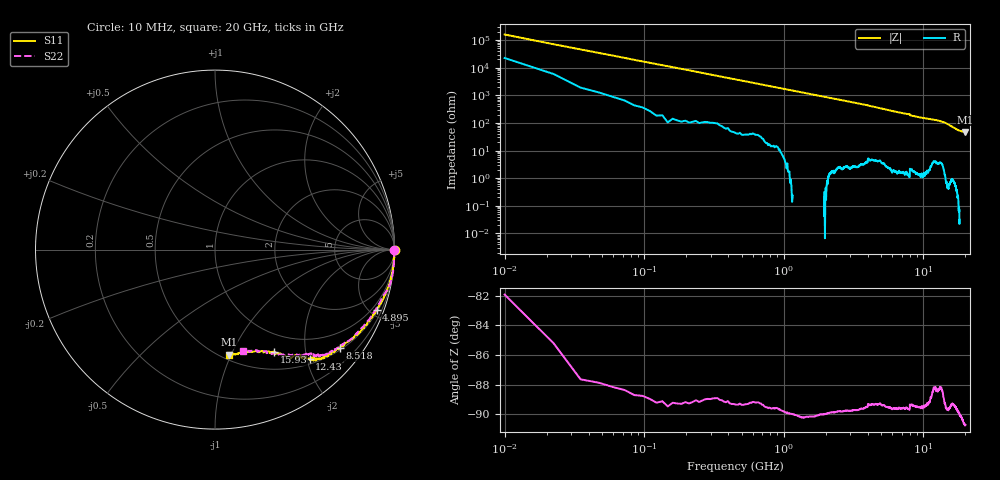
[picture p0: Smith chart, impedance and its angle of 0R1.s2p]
!Keysight Technologies,P5008B,MY61100088,A.16.20.02
!Date: Monday, May 27, 2024 12:57:32
!Correction: S11(C  2-Port  )
!S21(C  2-Port  )
!S12(C  2-Port  )
!S22(C  2-Port  )
!S2P File: Measurements: S11, S21, S12, S22:
# Hz S  dB  R 50
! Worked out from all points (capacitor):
!   1601 points, 10 MHz to 20 GHz, reference 50 ohm
!   read as one part in series: C = 94.1 fF near 110 MHz
!   lowest |Z| = 47.7 ohm at 20 GHz (marker M1)
!   S11 on the Smith chart (normalised r, x): 10 MHz: open; 4.895 GHz: 0.61, -5.43; 8.518 GHz: 0.56, -2.78; 12.43 GHz: 0.59, -2.05; 15.93 GHz: 0.73, -1.47; 20 GHz: 0.55, -0.98
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1e7  0.02 -0.0  -64.12 81.9  -64.26 81.7  -0.01 -0.0
1.349375e8  -0.01 -0.5  -41.89 88.6  -41.90 88.7  -0.01 -0.5
2.099e8  -0.01 -1.0  -38.17 88.4  -38.19 88.3  -0.01 -0.8
2.848625e8  0.00 -1.2  -35.50 87.8  -35.50 87.8  -0.01 -1.1
3.848125e8  -0.01 -1.4  -32.86 87.7  -32.87 87.7  -0.01 -1.5
6.721688e8  0.00 -2.6  -28.13 86.7  -28.15 86.7  -0.01 -2.5
1.10945e9  -0.02 -4.4  -23.88 85.8  -23.89 85.7  -0.00 -4.0
1.684162e9  -0.04 -6.7  -20.23 83.7  -20.25 83.7  -0.00 -6.1
2.4088e9  -0.05 -9.5  -17.23 80.5  -17.25 80.5  -0.02 -9.0
3.345831e9  -0.12 -13.4  -14.56 76.7  -14.57 76.7  -0.11 -12.6
4.895056e9  -0.34 -20.6  -11.15 69.4  -11.15 69.3  -0.36 -19.2
6.681662e9  -0.62 -28.7  -8.44 61.2  -8.46 61.3  -0.64 -27.8
7.893556e9  -0.78 -33.1  -7.47 56.9  -7.48 56.9  -0.81 -32.2
8.518244e9  -1.07 -38.3  -6.53 51.8  -6.53 51.9  -1.05 -36.6
1.0005e10  -1.34 -45.0  -5.67 46.0  -5.68 46.0  -1.36 -41.7
1.242879e10  -1.87 -49.1  -4.70 40.4  -4.71 40.4  -1.81 -46.6
1.334083e10  -2.13 -49.6  -4.20 39.0  -4.20 39.0  -2.14 -48.5
1.459021e10  -2.64 -55.2  -3.31 35.6  -3.32 35.7  -2.61 -52.0
1.592704e10  -3.64 -59.9  -2.42 28.1  -2.43 28.1  -3.59 -61.6
1.667666e10  -4.13 -66.0  -2.08 23.3  -2.09 23.4  -4.06 -65.4
1.82009e10  -4.55 -77.7  -1.78 14.5  -1.79 14.5  -4.52 -72.3
2e10  -4.57 -82.3  -1.69 11.2  -1.70 11.2  -4.62 -74.8
